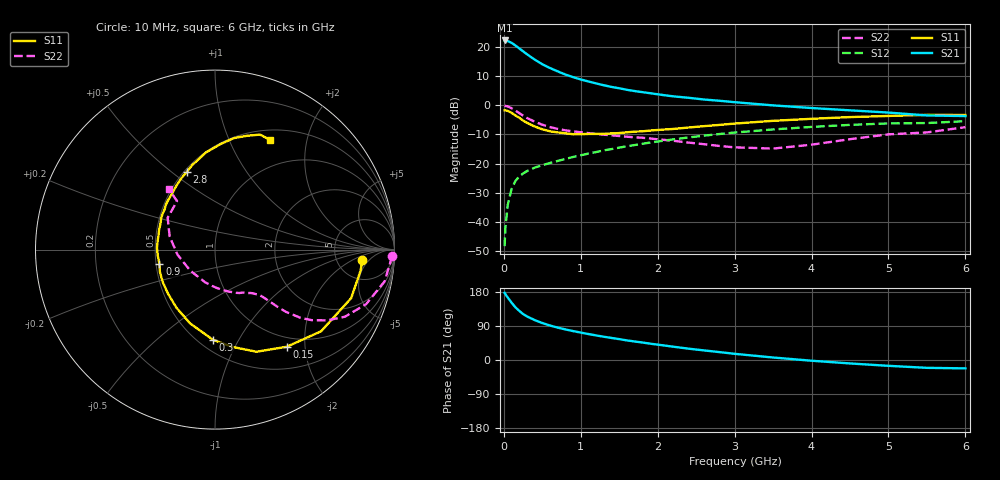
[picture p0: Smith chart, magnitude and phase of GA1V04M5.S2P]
! Infineon Technologies  Discrete & RF Semiconductors
! BF775
! Si NPN RF Bipolar Junction Transistor in SOT23
! VCE = 1 V  IC = 4.5 mA
! Common Emitter S-Parameters:  May  1996
# GHz  S  MA  R  50
!  f  S11  S21  S12  S22
! GHz  MAG  ANG  MAG  ANG  MAG  ANG  MAG  ANG
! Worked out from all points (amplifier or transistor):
!   36 points, 10 MHz to 6 GHz, reference 50 ohm
!   highest |S21| = 22.3 dB at 10 MHz (marker M1)
!   |S21| within 3 dB of that: start of sweep to 213.8 MHz
!   unconditionally stable (mu >= 1): 748.5 MHz to end of sweep
!   at 250 MHz: K = 0.48, MSG = 21.0 dB, |S12| = -23.4 dB
!   at 1.4 GHz: K = 1.18, MAG = 8.1 dB, |S12| = -15.0 dB
!   at 6 GHz: K = 1.04, MAG = -0.3 dB, |S12| = -5.4 dB
!   S11 on the Smith chart (normalised r, x): 10 MHz: 9.10, -3.33; 150 MHz: 0.84, -1.66; 300 MHz: 0.59, -0.79; 900 MHz: 0.52, -0.09; 2.8 GHz: 0.52, +0.57; 6 GHz: 0.62, +1.43
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0.01  0.8234 -4.1  13.09 177.2  0.0038 86.4  0.9868 -2.1
0.02  0.8195 -8.2  13.07 173.7  0.0078 84.4  0.979 -4.3
0.05  0.8056 -19.6  12.75 165.1  0.0193 79.4  0.9615 -10.6
0.1  0.7459 -37.6  11.94 151.5  0.0364 70.9  0.8956 -19.8
0.15  0.6727 -53.6  10.73 139.0  0.0502 63.0  0.8152 -27.3
0.2  0.6141 -67.9  9.565 129.8  0.0602 58.4  0.7395 -32.2
0.25  0.5494 -80.2  8.523 121.4  0.0676 54.8  0.6677 -36.1
0.3  0.5026 -91.3  7.594 115.0  0.0741 52.9  0.6088 -38.6
0.4  0.4341 -108.6  6.149 105.5  0.0851 50.6  0.5251 -41.3
0.5  0.3886 -123.6  5.098 97.5  0.0937 50.1  0.466 -42.6
0.6  0.3588 -136.9  4.395 91.0  0.1023 50.0  0.424 -43.4
0.7  0.3432 -147.7  3.849 85.5  0.111 50.6  0.3953 -44.1
0.9  0.3195 -165.6  3.062 76.3  0.1299 50.9  0.3579 -45.5
1.1  0.3234 178.3  2.578 68.5  0.1487 51.4  0.3338 -47.8
1.3  0.3246 165.7  2.221 61.4  0.1686 51.1  0.3134 -50.5
1.6  0.3452 150.5  1.855 51.7  0.1986 50.1  0.2894 -55.9
2.2  0.3938 127.3  1.432 35.2  0.2605 45.5  0.247 -71.6
2.8  0.462 109.7  1.203 20.9  0.3219 39.1  0.2012 -96.1
3.5  0.5434 95.4  1.001 6.6  0.3863 30.1  0.1811 -140.1
4.5  0.63 80.4  0.823 -9.1  0.4628 16.9  0.2629 163.9
5.5  0.688 68.6  0.672 -20.7  0.4978 3.0  0.3434 128.0
6  0.6843 63.5  0.656 -22.1  0.536 -0.9  0.4226 127.4
